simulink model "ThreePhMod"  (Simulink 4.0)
settings: Solver=ode23  StartTime=-eps  StopTime=0.02  FixedStep=0.000001  MaxStep=1e-5  RelTol=1e-3
undefined symbols (not defined in the file or in its folder): L, R, sfunxy, Sinus, Ts, Upp

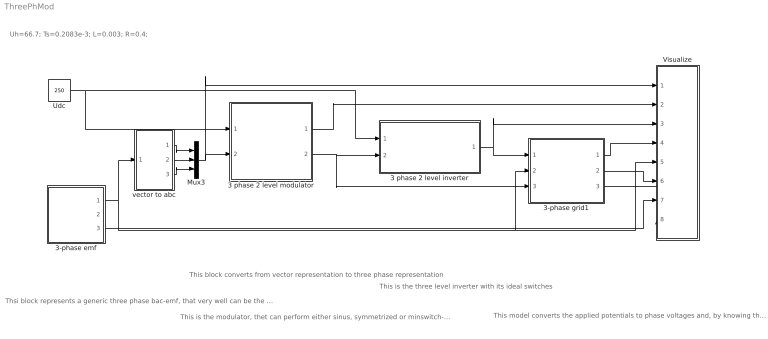
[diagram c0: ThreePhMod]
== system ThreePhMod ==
  note: Uh=66.7; Ts=0.2083e-3; L=0.003; R=0.4;
  note: Thsi block represents a generic three phase bac-emf, that very well can be the power line, having a 3-phase back-emf. In the same model, the back emf, the integral of the back emf (called "Psi") and the angle of the "Psi"- vetor is calculated. The three phase load model gives the output quantities in the alpha/beta reference frame, i.e. a vectors.
  note: This block converts from vector representation to three phase representation
  note: This is the modulator, thet can perform either sinus, symmetrized or minswitch- modulation with fixed or randomized carrier wave
  note: This is the three level inverter with its ideal switches
  note: This model converts the applied potentials to phase voltages and, by knowing the back-emf's it calculates the three phase currents. The phase voltages and phase currents are converted to vectors and serrved at the block output. The same block also calculates the DC link currents of the power electronic converter. This can be done if the switch positions and the phase currents are known. Hence, the switch position is supplied as input quantity.
  3 phase 2 level inverter : Subsystem  SimViewingDevice=off
  3 phase 2 level modulator : Subsystem  SimViewingDevice=off  mask{type=Sinus, Random=Fixed frequency, Ts=Ts}
      mask prompts: type "Sinus, Symmetrized or Minimum switch modulation"; Random "Fixed or random modulation?"; Ts "Sampling interval"
      mask help: Carrier Wave modulator that uses either fixed frequency modulation or random modulation. The fixed frequency modulation uses 1/(2Ts) as modulation frequency. The random modulation selects the modulatio frequency by random every sampling instant. The selection uses either 1/Ts, 1/(2Ts) or 1/(3Ts) as carrier wave frequency.
  3-phase emf : Subsystem  SimViewingDevice=off  mask{Upp=Upp, freq=50, Tc=0.1e-3}
      mask prompts: Upp "U_phase_to_phase [RMS]"; freq "Frequency"; Tc "Sampling time"
  3-phase grid1 : Subsystem  SimViewingDevice=off  mask{L=L, R=R}
      mask prompts: L "Inductance [H]"; R "Resistance [ohm]"
  Mux3 : Mux  Inputs=3
  Udc : Constant  Value=250
  Visualize : Subsystem  SimViewingDevice=off
  vector to abc : Subsystem  SimViewingDevice=off
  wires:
  Udc/1 -> 3 phase 2 level inverter/1(Udc), 3 phase 2 level modulator/1(Udc)
  3 phase 2 level modulator/2(sa,b,c) -> 3 phase 2 level inverter/2(sa,b,c), 3-phase grid1/3(s)
  3 phase 2 level modulator/1(mod) -> Visualize/2(mod)
  3 phase 2 level inverter/1(va,b,c) -> 3-phase grid1/1(va,b,c), Visualize/3(v)
  vector to abc/1(a) -> Mux3/1
  vector to abc/2(b) -> Mux3/2
  vector to abc/3(c) -> Mux3/3
  Mux3/1 -> 3 phase 2 level modulator/2(uabc*), Visualize/1(u*)
  3-phase emf/1(e_line) -> vector to abc/1(vect), 3-phase grid1/2(e_line), Visualize/5(e)
  3-phase grid1/1(u_ab) -> Visualize/4("u ")
  3-phase grid1/2(i_ab) -> Visualize/6(i)
  3-phase emf/3(Theta_line) -> Visualize/7(theta)
  3-phase grid1/3(i_dc) -> Visualize/8(idc)

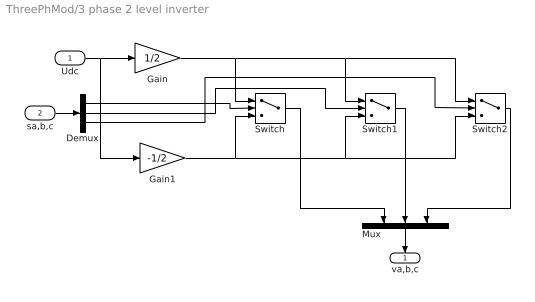
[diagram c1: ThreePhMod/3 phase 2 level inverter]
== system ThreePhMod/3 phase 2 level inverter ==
  Udc : Inport  Port=1  PortDimensions=-1  SampleTime=-1  DataType=auto
  sa,b,c : Inport  Port=2  PortDimensions=-1  SampleTime=-1  DataType=auto
  Demux : Demux  Outputs=3  BusSelectionMode=off
  Gain : Gain  Gain=1/2  Multiplication=Element-wise(K.*u)  SaturateOnIntegerOverflow=on
  Gain1 : Gain  Gain=-1/2  Multiplication=Element-wise(K.*u)  SaturateOnIntegerOverflow=on
  Mux : Mux  Orientation=down  Inputs=3
  Switch : Switch  Threshold=0
  Switch1 : Switch  Threshold=0
  Switch2 : Switch  Threshold=0
  va,b,c : Outport  Orientation=down  Port=1  InitialOutput=0
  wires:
  Gain/1 -> Switch/1, Switch1/1, Switch2/1
  Gain1/1 -> Switch/3, Switch1/3, Switch2/3
  Udc/1 -> Gain1/1, Gain/1
  sa,b,c/1 -> Demux/1
  Demux/1 -> Switch/2
  Demux/2 -> Switch1/2
  Demux/3 -> Switch2/2
  Switch/1 -> Mux/1
  Switch1/1 -> Mux/2
  Switch2/1 -> Mux/3
  Mux/1 -> va,b,c/1

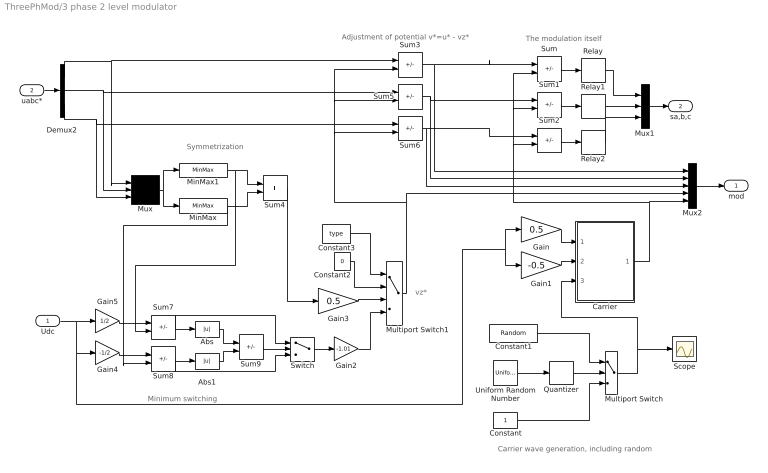
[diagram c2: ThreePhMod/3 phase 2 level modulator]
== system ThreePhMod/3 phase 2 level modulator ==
  note: Symmetrization
  note: vz*
  note: Minimum switching
  note: Carrier wave generation, including random
  note: Adjustment of potential v*=u* - vz*
  note: The modulation itself
  Udc : Inport  Port=1  PortDimensions=-1  SampleTime=-1  DataType=auto
  uabc* : Inport  Port=2  PortDimensions=-1  SampleTime=-1  DataType=auto
  Abs : Abs  SaturateOnIntegerOverflow=on
  Abs1 : Abs  SaturateOnIntegerOverflow=on
  Carrier : Subsystem  SimViewingDevice=off
  Constant : Constant  Value=1
  Constant1 : Constant  Value=Random
  Constant2 : Constant  Value=0
  Constant3 : Constant  Value=type
  Demux2 : Demux  Outputs=3  BusSelectionMode=off
  Gain : Gain  Gain=0.5  Multiplication=Element-wise(K.*u)  SaturateOnIntegerOverflow=on
  Gain1 : Gain  Gain=-0.5  Multiplication=Element-wise(K.*u)  SaturateOnIntegerOverflow=on
  Gain2 : Gain  Gain=-1.01  Multiplication=Element-wise(K.*u)  SaturateOnIntegerOverflow=on
  Gain3 : Gain  Gain=0.5  Multiplication=Element-wise(K.*u)  SaturateOnIntegerOverflow=on
  Gain4 : Gain  Gain=-1/2  Multiplication=Element-wise(K.*u)  SaturateOnIntegerOverflow=on
  Gain5 : Gain  Gain=1/2  Multiplication=Element-wise(K.*u)  SaturateOnIntegerOverflow=on
  MinMax : MinMax  Function=min  Inputs=1
  MinMax1 : MinMax  Function=max  Inputs=1
  Multiport Switch : MultiPortSwitch  Inputs=2
  Multiport Switch1 : MultiPortSwitch  Inputs=3
  Mux : Mux  Inputs=3
  Mux1 : Mux  Inputs=3
  Mux2 : Mux  Inputs=5
  Quantizer : Quantizer  QuantizationInterval=1  LinearizeAsGain=on
  Relay : Relay  OnSwitchValue=eps  OffSwitchValue=eps  OnOutputValue=1  OffOutputValue=-1
  Relay1 : Relay  OnSwitchValue=eps  OffSwitchValue=eps  OnOutputValue=1  OffOutputValue=-1
  Relay2 : Relay  OnSwitchValue=eps  OffSwitchValue=eps  OnOutputValue=1  OffOutputValue=-1
  Scope : Scope
  Sum{,1..3,5..8} (8 alike) : Sum  Inputs=+-  SaturateOnIntegerOverflow=on
  Sum4 : Sum  Inputs=++  SaturateOnIntegerOverflow=on
  Sum9 : Sum  Inputs=-+  SaturateOnIntegerOverflow=on
  Switch : Switch  Threshold=0
  Uniform Random Number : UniformRandomNumber  Minimum=1  Maximum=3  Seed=0.9874  SampleTime=Ts
  mod : Outport  Port=1  InitialOutput=0
  sa,b,c : Outport  Port=2  InitialOutput=0
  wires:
  Carrier/1(um) -> Sum2/2, Sum1/2, Sum/2, Mux2/5
  Gain1/1 -> Carrier/2(Umin)
  Gain/1 -> Carrier/1(Umax)
  Sum/1 -> Relay/1
  Relay1/1 -> Mux1/2
  Sum1/1 -> Relay1/1
  Relay2/1 -> Mux1/3
  Sum2/1 -> Relay2/1
  Quantizer/1 -> Multiport Switch/2
  Uniform Random Number/1 -> Quantizer/1
  Constant/1 -> Multiport Switch/3
  Multiport Switch/1 -> Carrier/3(x), Scope/1
  Constant1/1 -> Multiport Switch/1
  Sum3/1 -> Mux2/1, Sum/1
  Sum5/1 -> Mux2/2, Sum1/1
  Sum6/1 -> Mux2/3, Sum2/1
  Demux2/1 -> Sum3/1, Mux/1
  Demux2/2 -> Sum5/1, Mux/2
  Demux2/3 -> Sum6/1, Mux/3
  Mux/1 -> MinMax1/1, MinMax/1
  MinMax1/1 -> Sum4/1, Sum7/2
  MinMax/1 -> Sum4/2, Sum8/2
  Udc/1 -> Gain5/1, Gain4/1, Gain1/1, Gain/1
  Gain4/1 -> Sum8/1
  Sum7/1 -> Abs/1, Switch/1
  Sum8/1 -> Abs1/1, Switch/3
  Abs/1 -> Sum9/1
  Abs1/1 -> Sum9/2
  Sum9/1 -> Switch/2
  Sum4/1 -> Gain3/1
  Switch/1 -> Gain2/1
  Constant3/1 -> Multiport Switch1/1
  Constant2/1 -> Multiport Switch1/2
  Gain3/1 -> Multiport Switch1/3
  Gain2/1 -> Multiport Switch1/4
  Multiport Switch1/1 -> Sum5/2, Sum3/2, Sum6/2, Mux2/4
  Gain5/1 -> Sum7/1
  uabc*/1 -> Demux2/1
  Relay/1 -> Mux1/1
  Mux1/1 -> sa,b,c/1
  Mux2/1 -> mod/1

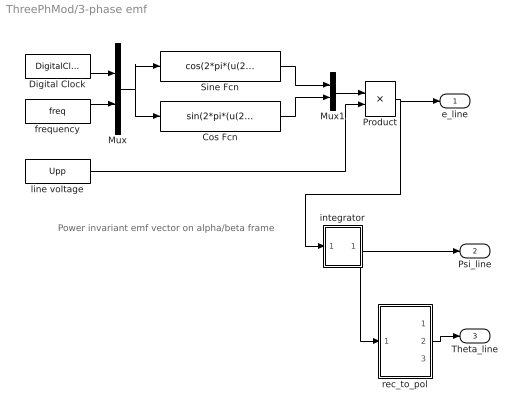
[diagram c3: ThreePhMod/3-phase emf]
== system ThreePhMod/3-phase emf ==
  note: Power invariant emf vector on alpha/beta frame
  Cos Fcn : Fcn  Expr=sin(2*pi*(u(2))*u(1)+pi/2)
  Digital Clock : DigitalClock  SampleTime=Tc
  Mux : Mux  Inputs=2
  Mux1 : Mux  Inputs=2
  Product : Product  Inputs=2  Multiplication=Element-wise(.*)  SaturateOnIntegerOverflow=on
  Sine Fcn : Fcn  Expr=cos(2*pi*(u(2))*u(1)+pi/2)
  frequency : Constant  Value=freq
  integrator : Subsystem  SimViewingDevice=off
  line voltage : Constant  Value=Upp
  rec_to_pol : Subsystem  SimViewingDevice=off
  e_line : Outport  Port=1  InitialOutput=0
  Psi_line : Outport  Port=2  InitialOutput=0
  Theta_line : Outport  Port=3  InitialOutput=0
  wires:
  Product/1 -> e_line/1, integrator/1(In1)
  Mux1/1 -> Product/1
  Cos Fcn/1 -> Mux1/2
  Sine Fcn/1 -> Mux1/1
  Mux/1 -> Cos Fcn/1, Sine Fcn/1
  Digital Clock/1 -> Mux/1
  frequency/1 -> Mux/2
  line voltage/1 -> Product/2
  integrator/1(Out1) -> Psi_line/1, rec_to_pol/1(rect)
  rec_to_pol/2(angle) -> Theta_line/1

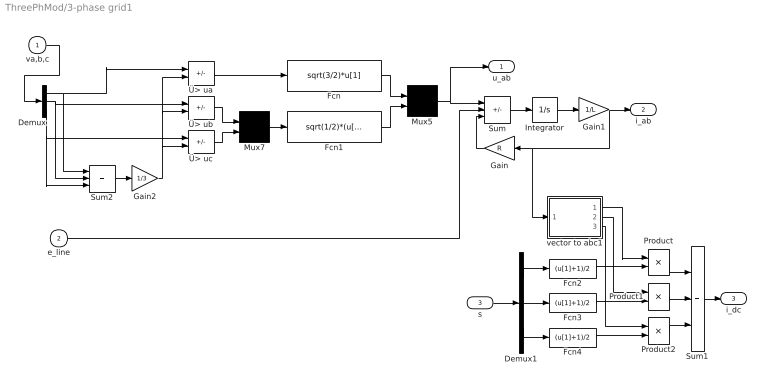
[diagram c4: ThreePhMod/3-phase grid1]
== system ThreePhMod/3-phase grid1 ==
  va,b,c : Inport  Port=1  PortDimensions=-1  SampleTime=-1  DataType=auto
  e_line : Inport  Port=2  PortDimensions=-1  SampleTime=-1  DataType=auto
  s : Inport  Port=3  PortDimensions=-1  SampleTime=-1  DataType=auto
  Demux : Demux  Outputs=3  BusSelectionMode=off
  Demux1 : Demux  Outputs=3  BusSelectionMode=off
  Fcn : Fcn  Expr=sqrt(3/2)*u[1]
  Fcn1 : Fcn  Expr=sqrt(1/2)*(u[1]-u[2])
  Fcn2 : Fcn  Expr=(u[1]+1)/2
  Fcn3 : Fcn  Expr=(u[1]+1)/2
  Fcn4 : Fcn  Expr=(u[1]+1)/2
  Gain : Gain  Orientation=left  Gain=R  Multiplication=Element-wise(K.*u)  SaturateOnIntegerOverflow=on
  Gain1 : Gain  Gain=1/L  Multiplication=Element-wise(K.*u)  SaturateOnIntegerOverflow=on
  Gain2 : Gain  Gain=1/3  Multiplication=Element-wise(K.*u)  SaturateOnIntegerOverflow=on
  Integrator : Integrator  ExternalReset=none  InitialConditionSource=internal  InitialCondition=0  LimitOutput=off  UpperSaturationLimit=inf  LowerSaturationLimit=-inf  ShowSaturationPort=off  ShowStatePort=off  AbsoluteTolerance=auto
  Mux5 : Mux  Inputs=2
  Mux7 : Mux  Inputs=2
  Product : Product  Inputs=2  Multiplication=Element-wise(.*)  SaturateOnIntegerOverflow=on
  Product1 : Product  Inputs=2  Multiplication=Element-wise(.*)  SaturateOnIntegerOverflow=on
  Product2 : Product  Inputs=2  Multiplication=Element-wise(.*)  SaturateOnIntegerOverflow=on
  Sum : Sum  Inputs=+--  SaturateOnIntegerOverflow=on
  Sum1 : Sum  Inputs=+++  SaturateOnIntegerOverflow=on
  Sum2 : Sum  Inputs=+++  SaturateOnIntegerOverflow=on
  vector to abc1 : Subsystem  SimViewingDevice=off
  Ü> ua : Sum  Inputs=+-  SaturateOnIntegerOverflow=on
  Ü> ub : Sum  Inputs=+-  SaturateOnIntegerOverflow=on
  Ü> uc : Sum  Inputs=+-  SaturateOnIntegerOverflow=on
  u_ab : Outport  Port=1  InitialOutput=0
  i_ab : Outport  Port=2  InitialOutput=0
  i_dc : Outport  Port=3
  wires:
  Gain1/1 -> i_ab/1, Gain/1, vector to abc1/1(vect)
  Integrator/1 -> Gain1/1
  Gain/1 -> Sum/3
  Sum/1 -> Integrator/1
  Fcn1/1 -> Mux5/2
  Fcn/1 -> Mux5/1
  Mux5/1 -> Sum/1, u_ab/1
  Mux7/1 -> Fcn1/1
  Ü> uc/1 -> Mux7/2
  Ü> ub/1 -> Mux7/1
  Ü> ua/1 -> Fcn/1
  Gain2/1 -> Ü> uc/2, Ü> ub/2, Ü> ua/2
  Demux/2 -> Ü> ub/1, Sum2/2
  Sum2/1 -> Gain2/1
  Demux/3 -> Ü> uc/1, Sum2/3
  Demux/1 -> Ü> ua/1, Sum2/1
  va,b,c/1 -> Demux/1
  Demux1/2 -> Fcn3/1
  Demux1/1 -> Fcn2/1
  Demux1/3 -> Fcn4/1
  s/1 -> Demux1/1
  Sum1/1 -> i_dc/1
  Product2/1 -> Sum1/3
  Product1/1 -> Sum1/2
  Product/1 -> Sum1/1
  vector to abc1/1(a) -> Product/1
  vector to abc1/2(b) -> Product1/1
  vector to abc1/3(c) -> Product2/1
  Fcn4/1 -> Product2/2
  Fcn3/1 -> Product1/2
  Fcn2/1 -> Product/2
  e_line/1 -> Sum/2

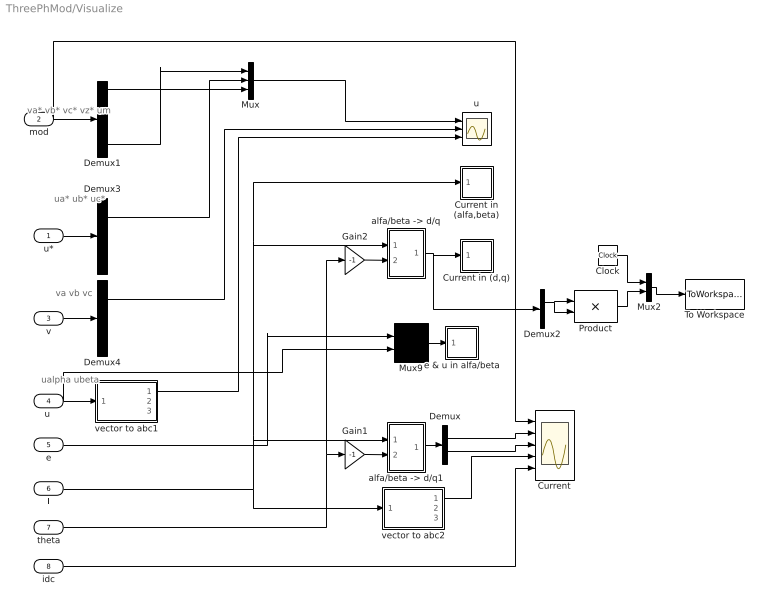
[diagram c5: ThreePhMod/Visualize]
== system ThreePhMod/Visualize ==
  note: va* vb* vc* vz* um
  note: ua* ub* uc*
  note: ualpha ubeta
  note: va vb vc
  u* : Inport  Port=1  PortDimensions=-1  SampleTime=-1  DataType=auto
  mod : Inport  Port=2  PortDimensions=-1  SampleTime=-1  DataType=auto
  v : Inport  Port=3  PortDimensions=-1  SampleTime=-1  DataType=auto
  "u " : Inport  Port=4  PortDimensions=-1  SampleTime=-1  DataType=auto
  e : Inport  Port=5  PortDimensions=-1  SampleTime=-1  DataType=auto
  i : Inport  Port=6  PortDimensions=-1  SampleTime=-1  DataType=auto
  theta : Inport  Port=7  PortDimensions=-1  SampleTime=-1  DataType=auto
  idc : Inport  Port=8  PortDimensions=-1  SampleTime=-1  DataType=auto
  Clock : Clock
  Current : Scope  NumInputPorts=5
  Current in (alfa,beta) : Subsystem  LoadFcn=sfunxy([],[],[],'LoadBlock')  StartFcn=sfunxy([],[],[],'Start')  StopFcn=sfunxy([],[],[],'Stop')  SimViewingDevice=off  mask(XY scope.){xmin=-5, xmax=5, ymin=-5, ymax=5, st=-1}
      mask prompts: xmin "x-min:"; xmax "x-max:"; ymin "y-min:"; ymax "y-max:"; st "Sample time:"
      mask help: XY scope using MATLAB graph window. First input is used as time base. Enter plotting ranges.
  Current in (d,q) : Subsystem  LoadFcn=sfunxy([],[],[],'LoadBlock')  StartFcn=sfunxy([],[],[],'Start')  StopFcn=sfunxy([],[],[],'Stop')  SimViewingDevice=off  mask(XY scope.){xmin=-5, xmax=5, ymin=-5, ymax=5, st=-1}
      mask prompts: xmin "x-min:"; xmax "x-max:"; ymin "y-min:"; ymax "y-max:"; st "Sample time:"
      mask help: XY scope using MATLAB graph window. First input is used as time base. Enter plotting ranges.
  Demux : Demux  Outputs=2  BusSelectionMode=off
  Demux1 : Demux  Outputs=5  BusSelectionMode=off
  Demux2 : Demux  Outputs=2  BusSelectionMode=off
  Demux3 : Demux  Outputs=3  BusSelectionMode=off
  Demux4 : Demux  Outputs=3  BusSelectionMode=off
  Gain1 : Gain  Gain=-1  Multiplication=Element-wise(K.*u)  SaturateOnIntegerOverflow=on
  Gain2 : Gain  Gain=-1  Multiplication=Element-wise(K.*u)  SaturateOnIntegerOverflow=on
  Mux : Mux  Inputs=3
  Mux2 : Mux  Inputs=2
  Mux9 : Mux  Inputs=2
  Product : Product  Inputs=2  Multiplication=Element-wise(.*)  SaturateOnIntegerOverflow=on
  To Workspace : ToWorkspace  VariableName=f1  SampleTime=-1  SaveFormat=Array
  "alfa/beta -> d/q" : Subsystem  SimViewingDevice=off
  "alfa/beta -> d/q1" : Subsystem  SimViewingDevice=off
  e & u in alfa/beta : Subsystem  LoadFcn=sfunxy([],[],[],'LoadBlock')  StartFcn=sfunxy([],[],[],'Start')  StopFcn=sfunxy([],[],[],'Stop')  SimViewingDevice=off  mask(XY scope.){xmin=-300, xmax=300, ymin=-300, ymax=300, st=-1}
      mask prompts: xmin "x-min:"; xmax "x-max:"; ymin "y-min:"; ymax "y-max:"; st "Sample time:"
      mask help: XY scope using MATLAB graph window. First input is used as time base. Enter plotting ranges.
  u : Scope  NumInputPorts=3
  vector to abc1 : Subsystem  SimViewingDevice=off
  vector to abc2 : Subsystem  SimViewingDevice=off
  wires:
  Gain2/1 -> "alfa/beta -> d/q"/2(angle)
  Gain1/1 -> "alfa/beta -> d/q1"/2(angle)
  "alfa/beta -> d/q1"/1(Out) -> Demux/1
  Demux/1 -> Current/2
  Demux/2 -> Current/3
  vector to abc2/1(a) -> Current/4
  mod/1 -> Demux1/1, Current/1
  "alfa/beta -> d/q"/1(Out) -> Current in (d,q)/1(xy), Demux2/1
  Demux1/5 -> Mux/1
  Demux1/1 -> Mux/3
  Mux/1 -> u/1
  u*/1 -> Demux3/1
  "u "/1 -> vector to abc1/1(vect), Mux9/2
  Demux3/1 -> Mux/2
  v/1 -> Demux4/1
  Demux4/1 -> u/2
  vector to abc1/1(a) -> u/3
  i/1 -> Current in (alfa,beta)/1(xy), "alfa/beta -> d/q"/1(vect), "alfa/beta -> d/q1"/1(vect), vector to abc2/1(vect)
  Mux9/1 -> e & u in alfa/beta/1(xy)
  e/1 -> Mux9/1
  theta/1 -> Gain1/1, Gain2/1
  Clock/1 -> Mux2/1
  Product/1 -> Mux2/2
  Mux2/1 -> To Workspace/1
  Demux2/1 -> Product/1, Product/2
  idc/1 -> Current/5

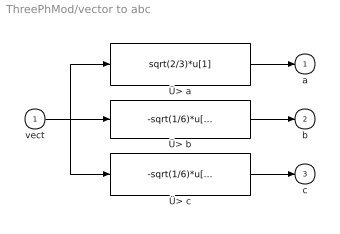
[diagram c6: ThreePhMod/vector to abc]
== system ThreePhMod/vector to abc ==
  vect : Inport  Port=1  PortDimensions=-1  SampleTime=-1  DataType=auto
  Ü> a : Fcn  Expr=sqrt(2/3)*u[1]
  Ü> b : Fcn  Expr=-sqrt(1/6)*u[1]+sqrt(1/2)*u[2]
  Ü> c : Fcn  Expr=-sqrt(1/6)*u[1]-sqrt(1/2)*u[2]
  a : Outport  Port=1  InitialOutput=0
  b : Outport  Port=2  InitialOutput=0
  c : Outport  Port=3  InitialOutput=0
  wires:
  vect/1 -> Ü> b/1, Ü> a/1, Ü> c/1
  Ü> b/1 -> b/1
  Ü> c/1 -> c/1
  Ü> a/1 -> a/1

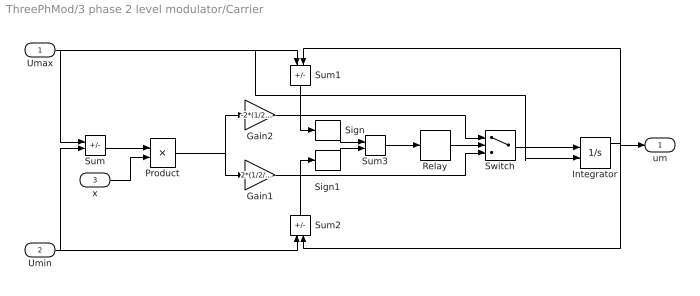
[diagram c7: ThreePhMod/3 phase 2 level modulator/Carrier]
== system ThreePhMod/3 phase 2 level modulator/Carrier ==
  Umax : Inport  Port=1  PortDimensions=-1  SampleTime=-1  DataType=auto
  Umin : Inport  Port=2  PortDimensions=-1  SampleTime=-1  DataType=auto
  x : Inport  Port=3  PortDimensions=-1  SampleTime=-1  DataType=auto
  Gain1 : Gain  Gain=2*(1/2/Ts)  Multiplication=Element-wise(K.*u)  SaturateOnIntegerOverflow=on
  Gain2 : Gain  Gain=-2*(1/2/Ts)  Multiplication=Element-wise(K.*u)  SaturateOnIntegerOverflow=on
  Integrator : Integrator  ExternalReset=none  InitialConditionSource=external  InitialCondition=0  LimitOutput=off  UpperSaturationLimit=inf  LowerSaturationLimit=-inf  ShowSaturationPort=off  ShowStatePort=off  AbsoluteTolerance=auto
  Product : Product  Inputs=2  Multiplication=Element-wise(.*)  SaturateOnIntegerOverflow=on
  Relay : Relay  OnSwitchValue=1  OffSwitchValue=-1  OnOutputValue=1  OffOutputValue=-1
  Sign : Signum
  Sign1 : Signum
  Sum : Sum  Inputs=+-  SaturateOnIntegerOverflow=on
  Sum1 : Sum  Orientation=down  Inputs=-+  SaturateOnIntegerOverflow=on
  Sum2 : Sum  Orientation=up  Inputs=-+  SaturateOnIntegerOverflow=on
  Sum3 : Sum  Inputs=++  SaturateOnIntegerOverflow=on
  Switch : Switch  Threshold=0
  um : Outport  Port=1
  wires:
  Switch/1 -> Integrator/1
  Umax/1 -> Sum/1, Sum1/1, Integrator/2
  Umin/1 -> Sum/2, Sum2/1
  Gain2/1 -> Switch/1
  Gain1/1 -> Switch/3
  Integrator/1 -> Sum1/2, um/1, Sum2/2
  Sum1/1 -> Sign/1
  Sum2/1 -> Sign1/1
  Sign/1 -> Sum3/1
  Sign1/1 -> Sum3/2
  Sum3/1 -> Relay/1
  Relay/1 -> Switch/2
  Sum/1 -> Product/1
  Product/1 -> Gain2/1, Gain1/1
  x/1 -> Product/2

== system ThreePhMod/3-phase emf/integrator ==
  note: Power invariant emf vector on alpha/beta frame
  In1 : Inport  Port=1  PortDimensions=-1  SampleTime=-1  DataType=auto
  Demux : Demux  Outputs=2  BusSelectionMode=off
  Integrator1 : Integrator  ExternalReset=none  InitialConditionSource=internal  InitialCondition=Upp/(2*pi*freq)  LimitOutput=off  UpperSaturationLimit=inf  LowerSaturationLimit=-inf  ShowSaturationPort=off  ShowStatePort=off  AbsoluteTolerance=auto
  Integrator2 : Integrator  ExternalReset=none  InitialConditionSource=internal  InitialCondition=0  LimitOutput=off  UpperSaturationLimit=inf  LowerSaturationLimit=-inf  ShowSaturationPort=off  ShowStatePort=off  AbsoluteTolerance=auto
  Mux : Mux  Inputs=2
  Out1 : Outport  Port=1
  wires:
  In1/1 -> Demux/1
  Mux/1 -> Out1/1
  Integrator2/1 -> Mux/2
  Integrator1/1 -> Mux/1
  Demux/2 -> Integrator2/1
  Demux/1 -> Integrator1/1

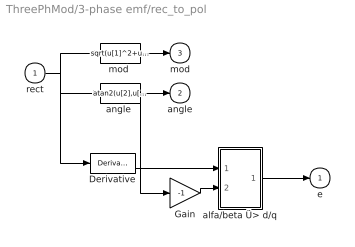
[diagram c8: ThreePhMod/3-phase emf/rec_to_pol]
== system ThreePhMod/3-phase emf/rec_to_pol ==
  rect : Inport  Port=1  PortDimensions=-1  SampleTime=-1  DataType=auto
  Derivative : Derivative
  Gain : Gain  Gain=-1  Multiplication=Element-wise(K.*u)  SaturateOnIntegerOverflow=on
  alfa/beta Ü> d/q : Subsystem  SimViewingDevice=off
  "angle " : Fcn  Expr=atan2(u[2],u[1])
  "mod " : Fcn  Expr=sqrt(u[1]^2+u[2]^2)
  e : Outport  Port=1  InitialOutput=0
  angle : Outport  Port=2  InitialOutput=0
  mod : Outport  Port=3  InitialOutput=0
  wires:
  "angle "/1 -> angle/1, Gain/1
  rect/1 -> "angle "/1, "mod "/1, Derivative/1
  "mod "/1 -> mod/1
  Gain/1 -> alfa/beta Ü> d/q/2(angle)
  Derivative/1 -> alfa/beta Ü> d/q/1(vect)
  alfa/beta Ü> d/q/1(Out) -> e/1

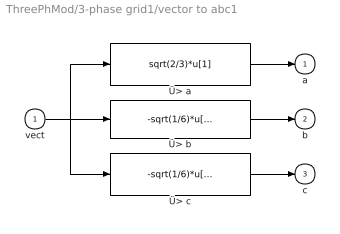
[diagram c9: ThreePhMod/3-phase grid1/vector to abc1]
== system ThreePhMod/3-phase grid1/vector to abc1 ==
  vect : Inport  Port=1  PortDimensions=-1  SampleTime=-1  DataType=auto
  Ü> a : Fcn  Expr=sqrt(2/3)*u[1]
  Ü> b : Fcn  Expr=-sqrt(1/6)*u[1]+sqrt(1/2)*u[2]
  Ü> c : Fcn  Expr=-sqrt(1/6)*u[1]-sqrt(1/2)*u[2]
  a : Outport  Port=1  InitialOutput=0
  b : Outport  Port=2  InitialOutput=0
  c : Outport  Port=3  InitialOutput=0
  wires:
  vect/1 -> Ü> b/1, Ü> a/1, Ü> c/1
  Ü> b/1 -> b/1
  Ü> c/1 -> c/1
  Ü> a/1 -> a/1

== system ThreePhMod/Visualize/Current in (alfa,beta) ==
  xy : Inport  Port=1  PortDimensions=-1  SampleTime=-1  DataType=auto
  sfunxy : S-Function  FunctionName=sfunxy  Parameters=[xmin xmax ymin ymax], st  PortCounts=[]  SFunctionModules=''
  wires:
  xy/1 -> sfunxy/1

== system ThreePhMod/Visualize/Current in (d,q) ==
  xy : Inport  Port=1  PortDimensions=-1  SampleTime=-1  DataType=auto
  sfunxy : S-Function  FunctionName=sfunxy  Parameters=[xmin xmax ymin ymax], st  PortCounts=[]  SFunctionModules=''
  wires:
  xy/1 -> sfunxy/1

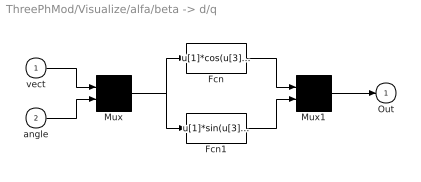
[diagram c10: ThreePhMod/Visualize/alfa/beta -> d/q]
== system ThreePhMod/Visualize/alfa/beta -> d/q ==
  vect : Inport  Port=1  PortDimensions=-1  SampleTime=-1  DataType=auto
  angle : Inport  Port=2  PortDimensions=-1  SampleTime=-1  DataType=auto
  Fcn : Fcn  Expr=u[1]*cos(u[3])-u[2]*sin(u[3])
  Fcn1 : Fcn  Expr=u[1]*sin(u[3])+u[2]*cos(u[3])
  Mux : Mux  Inputs=2
  Mux1 : Mux  Inputs=2
  Out : Outport  Port=1  InitialOutput=0
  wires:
  vect/1 -> Mux/1
  angle/1 -> Mux/2
  Mux/1 -> Fcn/1, Fcn1/1
  Fcn/1 -> Mux1/1
  Fcn1/1 -> Mux1/2
  Mux1/1 -> Out/1

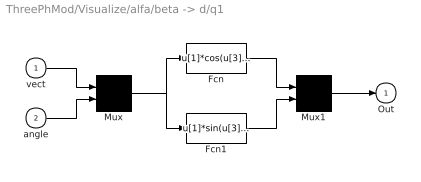
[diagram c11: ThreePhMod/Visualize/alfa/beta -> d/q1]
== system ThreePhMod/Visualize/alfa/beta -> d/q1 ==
  vect : Inport  Port=1  PortDimensions=-1  SampleTime=-1  DataType=auto
  angle : Inport  Port=2  PortDimensions=-1  SampleTime=-1  DataType=auto
  Fcn : Fcn  Expr=u[1]*cos(u[3])-u[2]*sin(u[3])
  Fcn1 : Fcn  Expr=u[1]*sin(u[3])+u[2]*cos(u[3])
  Mux : Mux  Inputs=2
  Mux1 : Mux  Inputs=2
  Out : Outport  Port=1  InitialOutput=0
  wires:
  Mux1/1 -> Out/1
  Fcn1/1 -> Mux1/2
  Fcn/1 -> Mux1/1
  Mux/1 -> Fcn1/1, Fcn/1
  angle/1 -> Mux/2
  vect/1 -> Mux/1

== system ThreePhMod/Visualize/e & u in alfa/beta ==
  xy : Inport  Port=1  PortDimensions=-1  SampleTime=-1  DataType=auto
  sfunxy : S-Function  FunctionName=sfunxy4  Parameters=[xmin xmax ymin ymax], st  PortCounts=[]  SFunctionModules=''
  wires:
  xy/1 -> sfunxy/1

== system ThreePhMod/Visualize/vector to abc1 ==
  vect : Inport  Port=1  PortDimensions=-1  SampleTime=-1  DataType=auto
  Ü> a : Fcn  Expr=sqrt(2/3)*u[1]
  Ü> b : Fcn  Expr=-sqrt(1/6)*u[1]+sqrt(1/2)*u[2]
  Ü> c : Fcn  Expr=-sqrt(1/6)*u[1]-sqrt(1/2)*u[2]
  a : Outport  Port=1  InitialOutput=0
  b : Outport  Port=2  InitialOutput=0
  c : Outport  Port=3  InitialOutput=0
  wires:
  Ü> a/1 -> a/1
  Ü> c/1 -> c/1
  Ü> b/1 -> b/1
  vect/1 -> Ü> c/1, Ü> a/1, Ü> b/1

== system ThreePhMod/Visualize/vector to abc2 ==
  vect : Inport  Port=1  PortDimensions=-1  SampleTime=-1  DataType=auto
  Ü> a : Fcn  Expr=sqrt(2/3)*u[1]
  Ü> b : Fcn  Expr=-sqrt(1/6)*u[1]+sqrt(1/2)*u[2]
  Ü> c : Fcn  Expr=-sqrt(1/6)*u[1]-sqrt(1/2)*u[2]
  a : Outport  Port=1  InitialOutput=0
  b : Outport  Port=2  InitialOutput=0
  c : Outport  Port=3  InitialOutput=0
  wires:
  vect/1 -> Ü> b/1, Ü> a/1, Ü> c/1
  Ü> b/1 -> b/1
  Ü> c/1 -> c/1
  Ü> a/1 -> a/1

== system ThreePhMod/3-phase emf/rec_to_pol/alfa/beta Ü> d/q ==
  vect : Inport  Port=1  PortDimensions=-1  SampleTime=-1  DataType=auto
  angle : Inport  Port=2  PortDimensions=-1  SampleTime=-1  DataType=auto
  Fcn : Fcn  Expr=u[1]*cos(u[3])-u[2]*sin(u[3])
  Fcn1 : Fcn  Expr=u[1]*sin(u[3])+u[2]*cos(u[3])
  Mux : Mux  Inputs=2
  Mux1 : Mux  Inputs=2
  Out : Outport  Port=1  InitialOutput=0
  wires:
  vect/1 -> Mux/1
  angle/1 -> Mux/2
  Mux/1 -> Fcn/1, Fcn1/1
  Fcn/1 -> Mux1/1
  Fcn1/1 -> Mux1/2
  Mux1/1 -> Out/1
